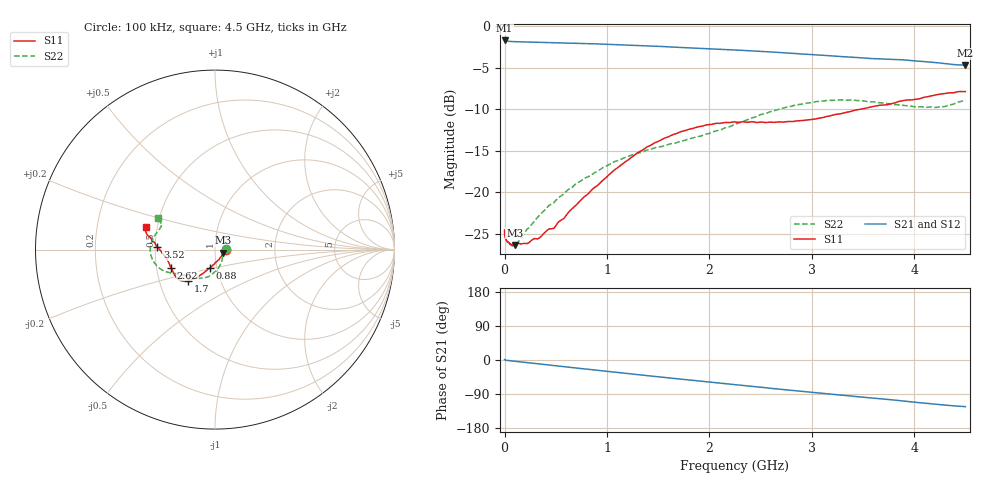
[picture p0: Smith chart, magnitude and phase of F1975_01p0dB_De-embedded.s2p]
! Integrated Device Technology
! Corporate Headquarters
! 6024 Silver Creek Valley Road
! San Jose, CA 95138  USA
! Phone:  1-408-284-8200
! Toll Free:  1-800-223-1366
! Webpage:  http://www.idt.com/
! Timing and RF Division
! 515 Groton Road, Suite 102
! Westford, MA 01886-6024
! Device:  F1975
! Description: 6-bit, 75 ohm, 0.5 dB Digital Step Attenuator
! Frequency:  5.0 MHz -  3.00 GHz
! Package:  4x4 mm QFN Plastic Package: 20 pin
! Ports:  2 RF, 11 DC
!  Pin  1  = D5 (16 dB)
!  Pin  2  = RF1  =  Port 1
!  Pin  3  = Serial Data In (DATA)
!  Pin  4  = Serial Clock (CLK)
!  Pin  5  = Serial Latch Enable (LE)
!  Pin  6  = VDD
!  Pin  7  = NC
!  Pin  8  = NC
!  Pin  9  = NC
!  Pin 10  = GND
!  Pin 11  = GND
!  Pin 12  = NC
!  Pin 13  = VMODE
!  Pin 14  = RF2  =  Port 2
!  Pin 15  = D4 (8 dB)
!  Pin 16  = D3 (4 dB)
!  Pin 17  = D2 (2 dB)
!  Pin 18  = NC
!  Pin 19  = D1 (1 dB)
!  Pin 20  = D0 (0.5 dB)
! State:  2
! Atten State:  1.0 dB
! Voltage:  +3.30 Volts
! Current:  0.593 mA
! Data:  The device was measured on a F1975 evaluation board which has
!  individual transmission lines to the RF pins.  Data was collected
!  using a calibrated network analyzer.  The evaluation board was
!  de-embedded using Automatic Fixture Removal (AFR).
!  The reference plane is the edge of the package pin.
! Misc:
!  Action Tracker AT0415
! Date Measured:  2018-02-08
! Date:  2018-03-26  MJV
! Note:
!  Integrated Device Technology supplies this data as a sample of measured
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# GHz S dB R 75
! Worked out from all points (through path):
!   291 points, 100 kHz to 4.5 GHz, reference 75 ohm
!   highest |S21| = -1.68 dB at 100 kHz (marker M1); lowest = -4.7 dB at 4.5 GHz (marker M2)
!   group delay of S21, straight-line fit = 77.2 ps
!   lowest |S11| = -26.3 dB at 100 MHz (marker M3), VSWR 1.10, Z = 82.1 - j2.78 ohm
!   |S11| at or under -10 dB: start of sweep to 3.461 GHz
!   |S22| runs from -26.5 to -8.8 dB; largest |S21 - S12| = 0.00024
!   S11 on the Smith chart (normalised r, x): 100 kHz: 1.13, +0.00; 880 MHz: 0.92, -0.19; 1.7 GHz: 0.70, -0.26; 2.62 GHz: 0.60, -0.13; 3.52 GHz: 0.51, +0.02; 4.5 GHz: 0.43, +0.13
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0.0001  -24.57 0.2  -1.68 1.2  -1.68 1.2  -24.41 0.8
0.0009  -25.08 -1.5  -1.72 1.0  -1.72 1.0  -24.97 -0.4
0.002  -25.30 -1.5  -1.73 0.8  -1.73 0.8  -25.14 -0.7
0.022  -25.85 -6.6  -1.77 -0.9  -1.77 -0.9  -25.88 -7.6
0.1  -26.31 -20.5  -1.83 -3.4  -1.83 -3.4  -26.36 -25.1
0.22  -26.15 -39.2  -1.87 -7.0  -1.87 -7.0  -24.40 -45.7
0.42  -24.51 -66.8  -1.93 -12.9  -1.93 -12.9  -21.74 -64.6
0.48  -24.33 -73.9  -1.95 -14.7  -1.95 -14.7  -21.25 -69.3
0.76  -20.73 -99.5  -2.05 -22.9  -2.05 -22.9  -18.47 -86.9
0.88  -19.37 -106.0  -2.09 -26.4  -2.09 -26.4  -17.60 -93.7
1.3  -15.21 -121.0  -2.29 -38.6  -2.29 -38.6  -15.24 -112.9
1.52  -13.72 -126.4  -2.40 -44.9  -2.40 -44.9  -14.48 -122.0
1.7  -12.79 -130.6  -2.52 -49.9  -2.51 -49.9  -13.90 -129.8
1.98  -11.85 -137.0  -2.68 -57.6  -2.68 -57.6  -12.92 -140.4
2.26  -11.51 -145.2  -2.84 -65.3  -2.84 -65.3  -11.75 -148.7
2.62  -11.55 -157.9  -3.08 -75.2  -3.08 -75.2  -10.18 -157.7
3.02  -11.17 -170.9  -3.40 -85.8  -3.40 -85.9  -9.12 -169.9
3.28  -10.51 -177.4  -3.61 -92.6  -3.61 -92.6  -8.85 -179.4
3.52  -9.86 177.2  -3.80 -98.7  -3.80 -98.7  -8.99 172.8
3.76  -9.37 173.2  -3.95 -104.6  -3.95 -104.6  -9.33 165.6
4.22  -8.21 167.4  -4.35 -117.0  -4.35 -117.0  -9.74 154.9
4.5  -7.85 162.0  -4.66 -123.2  -4.65 -123.2  -8.81 151.0
